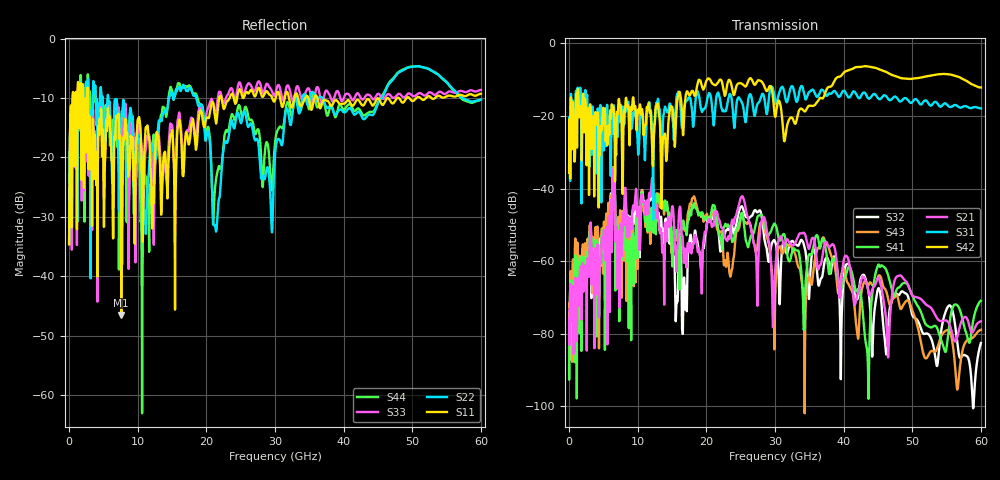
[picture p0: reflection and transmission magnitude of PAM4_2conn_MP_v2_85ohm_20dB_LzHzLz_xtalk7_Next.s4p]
! Info: Touchstone file created by Circ.  Input file=FAB50GbE_2conn_Midplane_Examax_Topo2_v2_85ohm_20dB_LzHzLz.circ
# Hz S RI R 50
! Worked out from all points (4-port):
!   6000 points, 10 MHz to 60 GHz, reference 50 ohm
!   strongest paths, dB at 10 MHz, 15.01 GHz, 30.01 GHz, 45.01 GHz, 60 GHz:
!     S42: -35.6, -17.4, -20.2, -7.0, -12.1
!     S31: -35.4, -19.6, -15.7, -15.1, -17.9
!     S21: -75.7, -45.2, -63.0, -64.5, -76.5
!     S41: -88.7, -58.8, -49.8, -61.1, -70.9
!     S43: -77.4, -55.1, -71.7, -64.3, -78.9
!     S32: -81.8, -54.1, -54.6, -67.6, -82.5
!   lowest |S11| = -46.5 dB at 7.61 GHz (marker M1), VSWR 1.01, Z = 49.6 + j0.15 ohm
!   |S11| at or under -10 dB: 2.767 GHz to 21.88 GHz (19.11 GHz wide, 155 % of centre); 22.2 GHz to 23.4 GHz (1.194 GHz wide, 5.24 % of centre); 36.17 GHz to 47.81 GHz (11.64 GHz wide, 27.7 % of centre)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
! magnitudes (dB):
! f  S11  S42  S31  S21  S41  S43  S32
! 10 MHz  -34.6  -35.6  -35.4  -75.7  -88.7  -77.4  -81.8
! 7.61 GHz  -46.5  -19.8  -17.4  -52.8  -55.2  -53.8  -52.8
! 12.2 GHz  -27.7  -33.2  -34.6  -37.6  -47.1  -45.7  -38.8
! 16.71 GHz  -22.1  -22.8  -18.6  -60.0  -49.4  -49.8  -65.4
! 25.22 GHz  -9.7  -11.2  -16.4  -42.1  -46.8  -47.5  -44.9
! 29.75 GHz  -10.4  -15.6  -12.8  -75.7  -50.1  -67.8  -54.3
! 60 GHz  -9.3  -12.1  -17.9  -76.5  -70.9  -78.9  -82.5
